[IBIS Ver]   3.2
[File Name]   sprm427.ibs
[File Rev]   1.0
[Date]   February 11, 2008
[Source]   File originated at Texas Instruments
[Copyright]   (c) 2008, Texas Instruments Inc.
[Component]   f28x3xzjz
[Manufacturer] Texas Instruments
[Package]
| Variable   Typ   Min   Max
R_pkg   0.252   0.219   0.435
L_pkg   4.0e-09   2.93e-09   8.99e-09
C_pkg   1.1e-12   0.8708e-12   2.7834e-12
[Pin] signal_name   model_name   R_pin   L_pin   C_pin
C2   GPIO30   BC3325CFHYPU   0.238  3.488e-09  0.969e-12
C1   GPIO29   BC3325CFHYPU   0.249  3.859e-09  0.928e-12
D1   GPIO0   BC3350AFHYPU   0.262  4.000e-09   0.929e-12
D2   GPIO1   BC3350AFHYPU   0.247  3.868e-09  0.988e-12
D3   GPIO2   BC3350AFHYPU   0.259  3.651e-09  1.216e-12
E1   GPIO3   BC3350AFHYPU   0.258  3.945e-09   0.931e-12
E2   GPIO4   BC3350AFHYPU   0.250   4.013e-09  1.006e-12
E3   GPIO5   BC3350AFHYPU   0.239   3.157e-09  1.059e-12
F1   GPIO6   BC3350AFHYPU   0.256  4.058e-09  0.956e-12
F2   GPIO7   BC3350AFHYPU   0.225  3.541e-09  0.932e-12
F3   GPIO8   BC3350AFHYPU   0.241  3.375e-09  1.165e-12
G1   GPIO9   BC3350AFHYPU   0.237  3.652e-09  0.912e-12
G2   GPIO10   BC3350AFHYPU   0.223  3.332e-09  0.904e-12
G3   GPIO11   BC3350AFHYPU   0.225   3.132e-09  1.090e-12
H1   GPIO12   BC3350AFHYPU   0.238  3.740e-09   0.924e-12
H2   GPIO13   BC3350AFHYPU   0.247  4.476e-09  1.119e-12
H3   GPIO14   BC3350AFHYPU   0.225  3.032e-09  1.045e-12
J1   GPIO15   BC3350AFHYPU   0.244   3.925e-09  0.976e-12
J2   GPIO16   BC3350AFHYPU   0.231   3.585e-09  1.011e-12
J3   GPIO17   BC3350AFHYPU   0.227  3.065e-09  1.099e-12
K3   VDD1A18   NC   0.227  3.340e-09  1.169e-12
K4   VDDA2   NC   0.241  4.128e-09  1.294e-12
K1   ADCINA7   NC   0.243  3.889e-09  0.890e-12
K2   ADCINA6   NC   0.258  4.765e-09  1.052e-12
L1   ADCINA5   NC   0.245  3.693e-09  0.955e-12
L2   ADCINA4   NC   0.257  4.909e-09  1.187e-12
L3   ADCINA3   NC   0.257  3.558e-09  1.233e-12
M1   ADCINA2   NC   0.253  4.019e-09  0.998e-12
M2   ADCINA1   NC   0.259  4.050e-09  1.757e-12
M3   ADCINA0   NC   0.249  3.501e-09  1.229e-12
N2   ADCLO   NC   0.268  4.07e-09   1.286e-12
L5   VDDAIO   NC   0.247  4.64e-09   1.3e-12
P3   ADCINB0   NC   0.249  3.921e-09  1.0e-12
N3   ADCINB1   NC   0.259  3.914e-09  1.127e-12
M4   ADCINB2   NC   0.226  3.066e-09  1.028e-12
N4   ADCINB3   NC   0.225  3.440e-09   1.0e-12
M5   ADCINB4   NC   0.223  2.930e-09  1.0e-12
N5   ADCINB5   NC   0.221  3.279e-09  1.0e-12
M6   ADCINB6   NC   0.232  3.290e-09  1.123e-12
N6   ADCINB7   NC   0.225  3.473e-09  1.0e-12
P7   ADCREFIN   NC   0.268  4.070e-09   1.286e-12
P4   ADCREFM   NC   0.345  4.524e-09  1.023e-12
P5   ADCREFP   NC   0.249  4.157e-09  1.137e-12
P6   ADCRESEXT   NC   0.244  3.808e-09  1.060e-12
L6   VDD2A18   NC   0.237  3.809e-09  0.8e-12
N8   GPIO18   BC3350AFHYPU   0.222  3.388e-09  0.895e-12
M8   GPIO19   BC3350AFHYPU   0.231  3.059e-09  0.987e-12
P9   GPIO20   BC3350AFHYPU   0.241   3.6e-09   0.969e-12
N9   GPIO21   BC3350AFHYPU   0.232  3.36e-09   0.976e-12
M9   GPIO22   BC3350AFHYPU   0.244  3.31e-09   1.032e-12
P10   GPIO23   BC3350AFHYPU   0.258   4.09e-09 0.992e-12
N10  GPIO24   BC3350AFHYPU   0.248  3.991e-09  1.033e-12
M10  GPIO25   BC3350AFHYPU   0.258  3.558e-09  0.985e-12
P11   GPIO26   BC3350AFHYPU   0.268  4.347e-09  1.014e-12
N11  GPIO27   BC3350AFHYPU   0.260  4.275e-09  1.032e-12
M11  GPIO32   BC3350AFHYPU   0.276  3.91e-09   1.35e-12
P12  GPIO33   BC3350AFHYPU   0.281  4.656e-09  0.94e-12
N12  TDI   IC33FFSHYPU   0.1989  8.731e-09  1.548e-12
N13  TDO   OC3325CF   0.345  6.245e-09  1.29e-12
L11  TRSTN   IC33FFSHYPD   0.342  5.8e-09   1.62e-12
M12  TMS   IC33FFSHYPU   0.312  4.533e-09   1.25e-12
M13  XRSN   BC3350BFODHYPU  0.352  6.4e-09   1.322e-12
M7  TEST1   NC   0.2027  3.139e-09  1.641e-12
L7   TEST2   NC   0.2047  3.255e-09  1.665e-12
L9   VDD3VFL   NC   0.2031  9.409e-09  1.689e-12
N7   EMU0   BC3325CFHYPU   0.371   7.422e-09  1.6757e-12
P8   EMU1   BC3325CFHYPU   0.396   8.501e-09  1.6201e-12
M14   TCK   IC33FFSHYPU   0.314   4.619e-09  1.01e-12
L14  GPIO48   BC3325CFHYPU   0.313  4.876e-09  1.1489e-12
L13  GPIO49   BC3325CFHYPU   0.251  3.905e-09  1.0e-12
L12  GPIO50   BC3325CFHYPU   0.241  3.3662e-09  1.1e-12
K14  GPIO51   BC3325CFHYPU   0.241  3.8558e-09  1.0e-12
K13   GPIO52   BC3325CFHYPU   0.227 3.708e-09  1.1e-12
K12  GPIO53   BC3325CFHYPU   0.224  3.182e-09  1.07e-12
J14  GPIO54   BC3325CFHYPU   0.231  3.671e-09  1.0e-12
J13  GPIO55   BC3325CFHYPU   0.224  3.6e-09   1.0e-12
J12  GPIO56   BC3325CFHYPU   0.224  2.88e-09   1.1e-12
H13  GPIO57   BC3325CFHYPU   0.228  3.5794e-09  0.93e-12
H12  GPIO58   BC3325CFHYPU   0.242   3.91e-09   1.1e-12
H14  X2   NC   0.241   3.79e-09  1.29e-12
G14  X1   NC   0.242   3.9e-09  0.9489e-12
G13  XCLKIN   IC33FFSHY   0.1948  8.424e-09  1.468e-12
H11  GPIO59   BC3325CFHYPU   0.224  4.0421e-09  1.16e-12
G12  GPIO60   BC3325CFHYPU   0.235  3.0429e-09  1.0e-12
F14  GPIO61   BC3325CFHYPU   0.249  3.976e-09  1.0e-12
F13  GPIO62   BC3325CFHYPU   0.2361 3.573e-09  1.03e-12
F12  GPIO63   BC3325CFHYPU   0.246  3.538e-09  1.142e-12
E14  GPIO64   BC3325CFHYPU   0.251  3.866e-09  1.0e-12
E13  GPIO65   BC3325CFHYPU   0.244  3.68e-09   0.976 e-12
E12  GPIO66   BC3325CFHYPU   0.247  3.446e-09  0.98e-12
D14  GPIO67   BC3325CFHYPU   0.255  4.073e-09  0.983e-12
D13  GPIO68   BC3325CFHYPU   0.25   3.967e-09  1.09e-12
D12  GPIO69   BC3325CFHYPU   0.255  3.571e-09  0.9e-12
C14  GPIO70   BC3325CFHYPU   0.265  4.178e-09  0.994e-12
C13  GPIO71   BC3325CFHYPU   0.269  4.34e-09  1.144e-12
B13  GPIO72   BC3325CFHYPU   0.279  4.48e-09  1.207e-12
A12  GPIO73   BC3325CFHYPU   0.283  4.501e-09  1.22e-12
B12  GPIO74   BC3325CFHYPU   0.287  4.19e-09  1.2e-12
C12  GPIO75   BC3325CFHYPU   0.263  3.76e-09  1.171e-12
A11  GPIO76   BC3325CFHYPU   0.239  3.755e-09  0.946e-12
B11  GPIO77   BC3325CFHYPU   0.221  3.432e-09  0.929e-12
C11  GPIO78   BC3325CFHYPU   0.236   3.558e-09  1.38e-12
B10  GPIO79   BC3325CFHYPU   0.220  3.473e-09  0.962e-12
C10  GPIO38   BC3325CFHYPU   0.223  3.066e-09   1.024e-12
A10  XCLKOUT   BC3325CF   0.235  3.58e-09   0.92e-12
D10  GPIO28   BC3325CFHYPU   0.232  3.77e-09  1.1e-12
A9  GPIO34   BC3350AFHYPU   0.238  3.88e-09   0.922e-12
C9  GPIO36   BC3325CFHYPU   0.226  3.206e-09  1.041e-12
B9  GPIO35   BC3325CFHYPU   0.233  3.4069e-09  0.89e-12
A8  XRDN   BC3325CFHYPU   0.236  3.988e-09  0.934e-12
B8  GPIO37   BC3325CFHYPU   0.219  3.488e-09  0.872e-12
C8  GPIO40   BC3325CFHYPU   0.221  3.030e-09  1.042e-12
A7  GPIO41   BC3325CFHYPU   0.235   3.346e-09  0.95e-12
B7  GPIO42   BC3325CFHYPU   0.225  3.6e-09   0.9711e-12
C7  GPIO43   BC3325CFHYPU   0.236  3.376e-09  1.0712e-12
A6  GPIO44   BC3325CFHYPU   0.257  4.121e-09  1.043e-12
B6  GPIO45   BC3325CFHYPU   0.238  3.98e-09  0.97e-12
C6  GPIO46   BC3325CFHYPU   0.234  3.242e-09  1.0493e-12
D6  GPIO47   BC3325CFHYPU   0.234  3.61e-09   1.175e-12
A5  GPIO80   BC3325CFHYPU   0.245  4.0156e-09  0.9517e-12
B5  GPIO81   BC3325CFHYPU   0.231  3.431e-09  0.92e-12
C5  GPIO82   BC3325CFHYPU   0.229  3.047e-09  0.92e-12
A4  GPIO83   BC3325CFHYPU   0.245  4.001e-09  0.96e-12
B4  GPIO84   BC3325CFHYPU   0.229  3.669e-09  0.981e-12
C4  GPIO85   BC3325CFHYPU   0.241  3.479e-09  1.022e-12
A3  GPIO86   BC3325CFHYPU   0.244  3.899e-09  0.963e-12
B3  GPIO87   BC3325CFHYPU   0.231  3.827e-09  1.033e-12
C3  GPIO39   BC3325CFHYPU   0.256  3.719e-09  1.32e-12
B2  GPIO31   BC3325CFHYPU   0.248  4.076e-09  1.089e-12
[Define Package Model]  f28x3xzjz
[Manufacturer]   ti
[OEM]   xyz
[Description]   f28x3x zjz
[Number Of Pins]   133
[Pin Numbers]
N3   | 1   N3   net1
L5   | 2   L5   net31
N4   | 3   N4   net20
P3   | 4   P3   net5
M4   | 5   M4   net2
N5   | 6   N5   net26
M5   | 7   M5   net37
N6   | 8   N6   net3
P7   | 9   P7   net23
M6   | 10   M6   net34
P6   | 11   P6   net11
P5   | 12   P5   net7
A14   | 13   A14   net4
P4   | 14   P4   net8
P8   | 15   P8   net6
M13   | 16   M13   net24
N12   | 17   N12   net12
L9   | 18   L9   net18
N13   | 19   N13   net10
P12   | 20   P12   net16
L4   | 21   L4   net9
N8   | 22   N8   net21
P9   | 23   P9   net13
N9   | 24   N9   net22
P10   | 25   P10   net14
N10   | 26   N10   net28
M8   | 27   M8   net41
P11   | 28   P11   net15
N11   | 29   N11   net29
L7   | 30   L7   net19
M7   | 31   M7   net17
N7   | 32   N7   net33
M12   | 33   M12   net45
M11   | 34   M11   net30
M10   | 35   M10   net43
M9   | 36   M9   net42
L6   | 37   L6   net36
M14   | 38   M14   net38
N2   | 39   N2   net25
M2   | 40   M2   net35
M1   | 41   M1   net39
M3   | 42   M3   net40
L2   | 43   L2   net49
A13   | 44   A13   net27
L11   | 45   L11   net32
L12   | 46   L12   net51
L13   | 47   L13   net48
L3   | 48   L3   net46
L14   | 49   L14   net47
L1   | 50   L1   net50
K4   | 51   K4   net54
D9   | 52   D9   net44
K14   | 53   K14   net57
K13   | 54   K13   net55
K2   | 55   K2   net52
K1   | 56   K1   net53
K12   | 57   K12   net56
J1   | 58   J1   net60
J2   | 59   J2   net61
H2   | 60   H2   net69
K3   | 61   K3   net58
J13   | 62   J13   net65
J14   | 63   J14   net63
J12   | 64   J12   net59
J3   | 65   J3   net62
H3   | 66   H3   net70
H12   | 67   H12   net64
H13   | 68   H13   net67
H1   | 69   H1   net68
G3   | 70   G3   net77
H14   | 71   H14   net66
H11   | 72   H11   net73
G12   | 73   G12   net74
G14   | 74   G14   net71
G13   | 75   G13   net72
G2   | 76   G2   net76
G1   | 77   G1   net75
F14   | 78   F14   net79
F13   | 79   F13   net78
F12   | 80   F12   net83
F2   | 81   F2   net81
F1   | 82   F1   net80
F3   | 83   F3   net82
E14   | 84   E14   net84
E13   | 85   E13   net85
E2   | 86   E2   net87
E1   | 87   E1   net86
E3   | 88   E3   net88
E12   | 89   E12   net89
D14   | 90   D14   net91
D13   | 91   D13   net90
D2   | 92   D2   net93
D1   | 93   D1   net92
C1   | 94   C1   net98
D12   | 95   D12   net97
C14   | 96   C14   net107
C2   | 97   C2   net99
D3   | 98   D3   net94
C3   | 99   C3   net100
D6   | 100   D6   net95
C6   | 101   C6   net111
C5   | 102   C5   net102
B5   | 103   B5   net124
B6   | 104   B6   net112
C7   | 105   C7   net103
D10   | 106   D10   net96
C9   | 107   C9   net105
C10   | 108   C10   net106
B10   | 109   B10   net123
B9   | 110   B9   net122
A9   | 111   A9   net134
C12   | 112   C12   net109
C13   | 113   C13   net108
B2   | 114   B2   net116
C4   | 115   C4   net101
B3   | 116   B3   net118
B4   | 117   B4   net119
B7   | 118   B7   net120
A6   | 119   A6   net130
C8   | 120   C8   net104
B8   | 121   B8   net113
C11   | 122   C11   net110
B11   | 123   B11   net114
B13   | 124   B13   net117
A12   | 125   A12   net121
B12   | 126   B12   net115
A5   | 127   A5   net126
A8   | 128   A8   net131
A11   | 129   A11   net133
A10   | 130   A10   net127
A3   | 131   A3   net129
A4   | 132   A4   net125
A7   | 133   A7   net132
[Model Data]
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[End Model Data]
[End Package Model]
| End of package information
|   Component BC3325CFHYPU
[Component]   BC3325CFHYPU
[Manufacturer]   Texas Instruments.
[Package]
| variable   typ   min   max
R_pkg   0.000   0.000   0.000
L_pkg   0.000H   0.000H   0.000H
C_pkg   0.000F   0.000F   0.000F
[Pin]  signal_name   model_name   R_pin   L_pin   C_pin
PAD   PAD   BC3325CFHYPU_3P3PU
| A   A   dummy
| GZ   GZ   dummy
| Y   Y   dummy
VSSS   VSSS   GND
VDDS   VDDS   POWER
[Model Selector]   BC3325CFHYPU
BC3325CFHYPU_2P5PU   cell  VDDS=2.75(TYP)  PI=0
BC3325CFHYPU_2P5PUZ   cell  VDDS=2.75(TYP)  PI=1
BC3325CFHYPU_3P3PU   cell  VDDS=3.3(TYP)  PI=0
BC3325CFHYPU_3P3PUZ   cell  VDDS=3.3(TYP)  PI=1
|   Component BC3350AFHYPU
[Component]   BC3350AFHYPU
[Manufacturer]   Texas Instruments.
[Package]
| variable   typ   min   max
R_pkg   0.000   0.000   0.000
L_pkg   0.000H   0.000H   0.000H
C_pkg   0.000F   0.000F   0.000F
[Pin]  signal_name   model_name   R_pin   L_pin   C_pin
PAD   PAD   BC3350AFHYPU_3P3PU
| A   A   dummy
| GZ   GZ   dummy
| Y   Y   dummy
VSSS   VSSS   GND
VDDS   VDDS   POWER
[Model Selector]  BC3350AFHYPU
BC3350AFHYPU_2P5PU   cell   VDDS=2.5V(typ)  PI=0
BC3350AFHYPU_2P5PUZ  cell   VDDS=2.5V(typ)  PI=1
BC3350AFHYPU_3P3PU   cell   VDDS=3.3V(typ)  PI=0
BC3350AFHYPU_3P3PUZ  cell   VDDS=3.3V(typ)  PI=1
|   Component OC3325CF
[Component]   OC3325CF
[Manufacturer]   Texas Instruments.
[Package]
| variable   typ   min   max
R_pkg   0.000   0.000   0.000
L_pkg   0.000H   0.000H   0.000H
C_pkg   0.000F   0.000F   0.000F
[Pin]  signal_name   model_name   R_pin   L_pin   C_pin
PAD   PAD   OC3325CF_3P3
| A   A   dummy
| GZ   GZ   dummy
VDDS   VDDS   POWER
VSSS   VSSS   GND
VSS   VSS   GND
[Model Selector]   OC3325CF
OC3325CF_2P5  cell VDDS=2.5V(typ)
OC3325CF_2P7  cell VDDS=2.75V(typ)
OC3325CF_3P3  cell VDDS=3.3V(typ)
|   Component IC33FFSHYPD
[Component]   IC33FFSHYPD
[Manufacturer]   Texas Instruments.
[Package]
| variable   typ   min   max
R_pkg   0.000   0.000   0.000
L_pkg   0.000H   0.000H   0.000H
C_pkg   0.000F   0.000F   0.000F
[Pin]  signal_name   model_name   R_pin   L_pin   C_pin
PAD   PAD   IC33FFSHYPD_3P3PD
| Y   Y   dummy
VSS   VSS   GND
VDDS   VDDS   POWER
[Model Selector]  IC33FFSHYPD
IC33FFSHYPD_2P7PD   cell with PI=0 and VDDS as 2.75(typ)
IC33FFSHYPD_2P7PDZ   cell with PI=1 and VDDS as 2.75(typ)
IC33FFSHYPD_3P3PD   cell with PI=0 and VDDS as 3.3(typ)
IC33FFSHYPD_3P3PDZ   cell with PI=1 and VDDS as 3.3(typ)
|   Component IC33FFSHYPU
[Component]   IC33FFSHYPU
[Manufacturer]   Texas Instruments.
[Package]
| variable   typ   min   max
R_pkg   0.000   0.000   0.000
L_pkg   0.000H   0.000H   0.000H
C_pkg   0.000F   0.000F   0.000F
[Pin]  signal_name   model_name   R_pin   L_pin   C_pin
PAD   PAD   IC33FFSHYPU_3P3PU
| Y   Y   dummy
VSS   VSS   GND
VDDS   VDDS   POWER
[Model Selector]  IC33FFSHYPU
IC33FFSHYPU_2P5PU   cell with PI=0 VDDS=2.5(typ)
IC33FFSHYPU_2P5PUZ   cell with PI=1 VDDS=2.5(typ)
IC33FFSHYPU_2P7PU   cell with PI=0 VDDS=2.7(typ)
IC33FFSHYPU_2P7PUZ   cell with PI=1 VDDS=2.7(typ)
IC33FFSHYPU_3P3PU   cell with PI=0 VDDS=3.3(typ)
IC33FFSHYPU_3P3PUZ   cell with PI=1 VDDS=3.3(typ)
|   Component BC3325CF
[Component]   BC3325CF
[Manufacturer]   Texas Instruments.
[Package]
| variable   typ   min   max
R_pkg   0.000   0.000   0.000
L_pkg   0.000H   0.000H   0.000H
C_pkg   0.000F   0.000F   0.000F
[Pin]  signal_name   model_name   R_pin   L_pin   C_pin
PAD   PAD   BC3325CF_3P3PU
| A   A   dummy
| GZ   GZ   dummy
| Y   Y   dummy
VSSS   VSSS   GND
VDDS   VDDS   POWER
[Model Selector]  BC3325CF
BC3325CF_2P5PU  cell   VDDS=2.75V(typ)
BC3325CF_3P3PU  cell   VDDS=3.30V(typ)
|   Component BC3350BFODHYPU
[Component]   BC3350BFODHYPU
[Manufacturer]   Texas Instruments.
[Package]
| variable   typ   min   max
R_pkg   0.000   0.000   0.000
L_pkg   0.000H   0.000H   0.000H
C_pkg   0.000F   0.000F   0.000F
[Pin]  signal_name   model_name   R_pin   L_pin   C_pin
PAD   PAD   BC3350BFODHYPU_3P3PU
| A   A   dummy
| GZ   GZ   dummy
| Y   Y   dummy
VSSS   VSSS   GND
VDDS   VDDS   POWER
[Model Selector]   BC3350BFODHYPU
BC3350BFODHYPU_2P5PU   cell   VDDS=2.75(TYP)
BC3350BFODHYPU_2P5PZ   cell   VDDS=2.75(TYP)
BC3350BFODHYPU_3P3PU   cell   VDDS=3.3(TYP)
BC3350BFODHYPU_3P3PZ   cell   VDDS=3.3(TYP)
|   Component IC33FFSHY
[Component]   IC33FFSHY
[Manufacturer]   Texas Instruments.
[Package]
| variable   typ   min   max
R_pkg   0.000   0.000   0.000
L_pkg   0.000H   0.000H   0.000H
C_pkg   0.000F   0.000F   0.000F
[Pin]  signal_name   model_name   R_pin   L_pin   C_pin
PAD   PAD   IC33FFSHY_3P3
| Y   Y   dummy
VSS   VSS   GND
VDDS   VDDS   POWER
[Model Selector]  IC33FFSHY
IC33FFSHY_2P5   cell with VDDS=2.5(NOM)
IC33FFSHY_2P7   cell with VDDS=2.7(NOM)
IC33FFSHY_3P3   cell with VDDS=3.3(NOM)
| Models and submodels in the file (30): BC3325CFHYPU_2P5PU (I/O), BC3325CFHYPU_2P5PUZ (I/O), BC3325CFHYPU_3P3PU (I/O), BC3325CFHYPU_3P3PUZ (I/O), BC3350AFHYPU_2P5PU (I/O), BC3350AFHYPU_2P5PUZ (I/O), BC3350AFHYPU_3P3PU (I/O), BC3350AFHYPU_3P3PUZ (I/O), OC3325CF_2P5 (3-state), OC3325CF_2P7 (3-state), OC3325CF_3P3 (3-state), IC33FFSHYPD_2P7PD (Input), IC33FFSHYPD_2P7PDZ (Input), IC33FFSHYPD_3P3PD (Input), IC33FFSHYPD_3P3PDZ (Input), IC33FFSHYPU_2P5PU (Input), IC33FFSHYPU_2P5PUZ (Input), IC33FFSHYPU_2P7PU (Input), IC33FFSHYPU_2P7PUZ (Input), IC33FFSHYPU_3P3PU (Input), IC33FFSHYPU_3P3PUZ (Input), BC3325CF_2P5PU (I/O), BC3325CF_3P3PU (I/O), BC3350BFODHYPU_2P5PU (I/O_open_drain), BC3350BFODHYPU_2P5PZ (I/O_open_drain), BC3350BFODHYPU_3P3PU (I/O_open_drain), BC3350BFODHYPU_3P3PZ (I/O_open_drain), IC33FFSHY_2P5 (Input), IC33FFSHY_2P7 (Input), IC33FFSHY_3P3 (Input)
